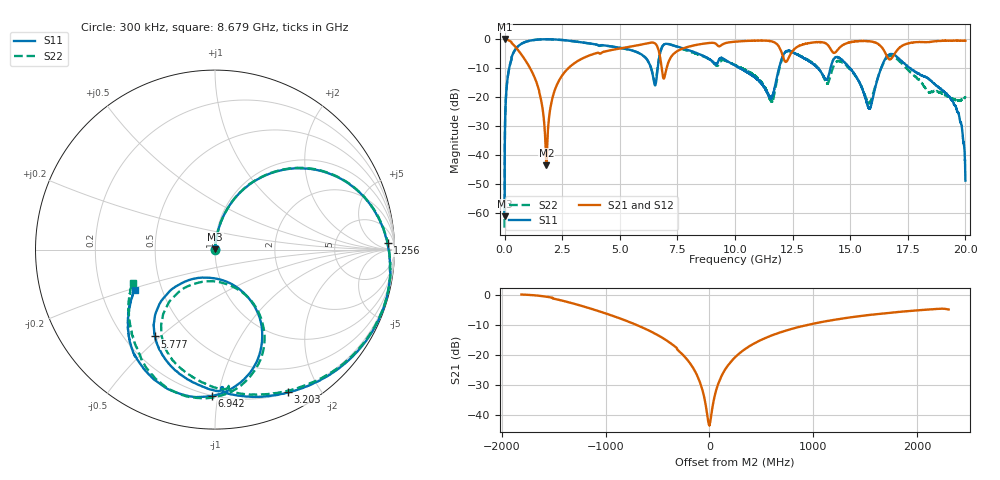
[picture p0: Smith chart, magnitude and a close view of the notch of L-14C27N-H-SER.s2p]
!{L-14C27N}
!Johanson Technology Inc.
!www.johansontechnology.com
!Test Board Conditions:
!Substrate Type  RO4350B
!Substrate Thickness  20 mil
!Substrate Dk  3.66
!TL Type: GCPW
!TL Trace Width  36 mil
!TL Gap  12 mil
!Electrode orientation  Horizontal
!DUT TOPOLOGY	SERIES
!Mounting Pad LxW  26x36 mil
! Created Sun Jun 20 13:03:52 2021
# hz S ma R 50
! 2 Port Network Data from SP1.SP block
! freq  magS11  angS11  magS21  angS21  magS12  angS12  magS22  angS22
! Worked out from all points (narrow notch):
!   20001 points, 300 kHz to 20 GHz, reference 50 ohm
!   highest |S21| = 0.00 dB at 6.3 MHz (marker M1); lowest = -43.5 dB at 1.812 GHz (marker M2)
!   notch at M2: 41.4 dB deep, 384 MHz wide at half that depth
!   lowest |S11| = -61.1 dB at 300 kHz (marker M3), VSWR 1.00, Z = 50.1 + j0.07 ohm
!   |S11| at or under -10 dB: 10.22 GHz to 11.91 GHz (1.691 GHz wide, 15.3 % of centre); 14.99 GHz to 16.34 GHz (1.355 GHz wide, 8.65 % of centre); 17.6 GHz to end of sweep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
!   |S22| runs from -65.0 to -0.1 dB; largest |S21 - S12| = 0.013
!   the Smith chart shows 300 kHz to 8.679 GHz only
!   S11 on the Smith chart (normalised r, x): 300 kHz: 1.00, +0.00; 1.256 GHz: 27, +26; 3.203 GHz: 0.20, -1.62; 5.777 GHz: 0.32, -0.48; 6.942 GHz: 0.20, -0.96; 8.679 GHz: 0.35, -0.21
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300000  0.0008785 52.7  0.9997 -0.1  0.9993 -0.1  0.0005621 57.4
6300000  0.01169 89.0  0.9998 -0.7  0.9997 -0.7  0.01196 88.9
1.073e8  0.1769 76.8  0.978 -11.2  0.9776 -11.2  0.1778 76.7
2.553e8  0.3917 63.4  0.9124 -25.5  0.912 -25.4  0.3931 63.5
1.2563e9  0.9621 2.1  0.2395 -85.8  0.2402 -85.9  0.9631 2.5
1.8123e9  0.9935 -17.7  0.006689 -13.9  0.006796 -13.6  0.9924 -16.9
2.2353e9  0.9826 -31.8  0.1509 56.1  0.151 56.1  0.9803 -30.6
3.2033e9  0.8935 -62.9  0.4249 27.1  0.4259 27.0  0.8933 -60.4
3.3343e9  0.8802 -66.9  0.4541 23.2  0.4552 23.2  0.8794 -64.2
5.7773e9  0.5885 -124.7  0.7812 -34.8  0.7815 -34.9  0.5882 -119.6
6.6673e9  0.3711 -55.0  0.6772 -93.4  0.6761 -93.3  0.3841 -54.6
6.9423e9  0.8152 -91.3  0.2227 -51.2  0.2224 -51.0  0.8206 -89.6
8.6793e9  0.4994 -153.4  0.8383 -69.2  0.838 -69.2  0.4944 -158.0
1.00003e10  0.3509 -179.3  0.902 -93.1  0.9041 -93.1  0.3576 -176.4
1.15803e10  0.09728 -151.7  0.9146 -134.3  0.9148 -134.3  0.08447 -159.6
1.22083e10  0.6101 -155.0  0.404 -133.5  0.4064 -134.0  0.5983 -150.5
1.33343e10  0.3875 139.2  0.8676 -136.4  0.864 -136.4  0.3962 141.7
1.45793e10  0.4564 134.5  0.7358 -144.8  0.7362 -144.8  0.4131 156.0
1.58303e10  0.06382 156.3  0.9172 178.4  0.9178 178.3  0.07887 180.0
1.66673e10  0.5313 165.3  0.4568 165.0  0.4511 165.7  0.5004 177.7
1.93883e10  0.08999 46.2  0.937 136.1  0.9398 136.1  0.0956 95.6
2e10  0.003641 70.8  0.9358 123.0  0.9306 123.0  0.1001 136.4
